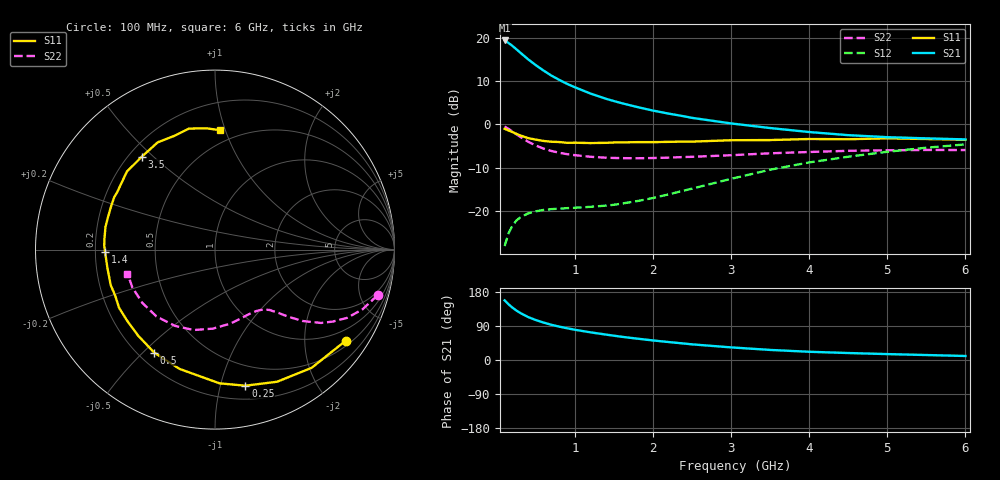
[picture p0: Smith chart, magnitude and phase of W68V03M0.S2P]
! SIEMENS Small Signal Semiconductors
! BFR193W
! Si NPN RF Bipolar Junction Transistor in SOT323
! VCE = 8 V  IC = 3 mA
! Common Emitter S-Parameters:  September  1992
# GHz  S  MA  R  50
!  f  S11  S21  S12  S22
! GHz  MAG  ANG  MAG  ANG  MAG  ANG  MAG  ANG
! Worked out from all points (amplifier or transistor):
!   28 points, 100 MHz to 6 GHz, reference 50 ohm
!   highest |S21| = 19.3 dB at 100 MHz (marker M1)
!   |S21| within 3 dB of that: start of sweep to 313 MHz
!   unconditionally stable (mu >= 1): 1.38 GHz to 2.62 GHz
!   at 300 MHz: K = 0.25, MSG = 19.0 dB, |S12| = -21.5 dB
!   at 1.5 GHz: K = 1.04, MAG = 10.8 dB, |S12| = -18.5 dB
!   at 6 GHz: K = 0.92, MSG = 0.6 dB, |S12| = -4.6 dB
!   S11 on the Smith chart (normalised r, x): 100 MHz: 0.64, -3.06; 250 MHz: 0.31, -1.20; 500 MHz: 0.26, -0.54; 1.4 GHz: 0.24, -0.01; 3.5 GHz: 0.25, +0.46; 6 GHz: 0.40, +0.96
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0.1  0.8878 -34.9  9.263 157.3  0.0394 71.1  0.9406 -15.7
0.15  0.8506 -50.8  8.661 147.0  0.0556 63.3  0.8862 -22.1
0.2  0.8136 -64.8  8.015 138.2  0.0678 57.1  0.8275 -27.4
0.25  0.777 -77.4  7.344 130.7  0.0777 51.5  0.7681 -31.5
0.3  0.7454 -88.1  6.709 124.2  0.0845 47.2  0.7178 -34.7
0.4  0.6935 -106.5  5.63 113.4  0.094 41.1  0.6313 -39.1
0.5  0.6664 -120.5  4.799 105.4  0.0994 37.4  0.5696 -41.7
0.6  0.643 -131.7  4.159 98.7  0.1032 35.4  0.5242 -43.8
0.7  0.6298 -141.0  3.64 92.9  0.1053 34.5  0.4931 -45.2
0.8  0.6251 -148.8  3.252 88.0  0.1067 34.4  0.4701 -46.8
0.9  0.6122 -155.3  2.926 83.8  0.1081 34.9  0.4528 -47.9
1  0.6138 -161.2  2.674 79.8  0.1092 35.9  0.4411 -49.5
1.2  0.6081 -170.6  2.263 73.0  0.1119 38.9  0.4226 -52.6
1.4  0.6123 -178.7  1.967 67.0  0.1157 43.0  0.4124 -56.2
1.8  0.6234 168.2  1.581 56.3  0.1305 52.4  0.4064 -64.2
2.2  0.6277 156.9  1.329 47.4  0.1557 60.0  0.4131 -72.8
2.5  0.6318 149.8  1.187 41.3  0.1814 63.8  0.422 -79.5
3  0.6557 138.5  1.024 33.3  0.2354 66.3  0.4406 -91.7
3.5  0.6587 128.4  0.906 26.6  0.2998 64.5  0.4637 -104.9
4.5  0.673 109.5  0.75 18.4  0.4231 55.4  0.4951 -131.2
5.5  0.6773 94.0  0.689 13.1  0.5375 44.3  0.5064 -155.3
6  0.666 87.4  0.67 10.6  0.5874 37.9  0.5055 -164.7
